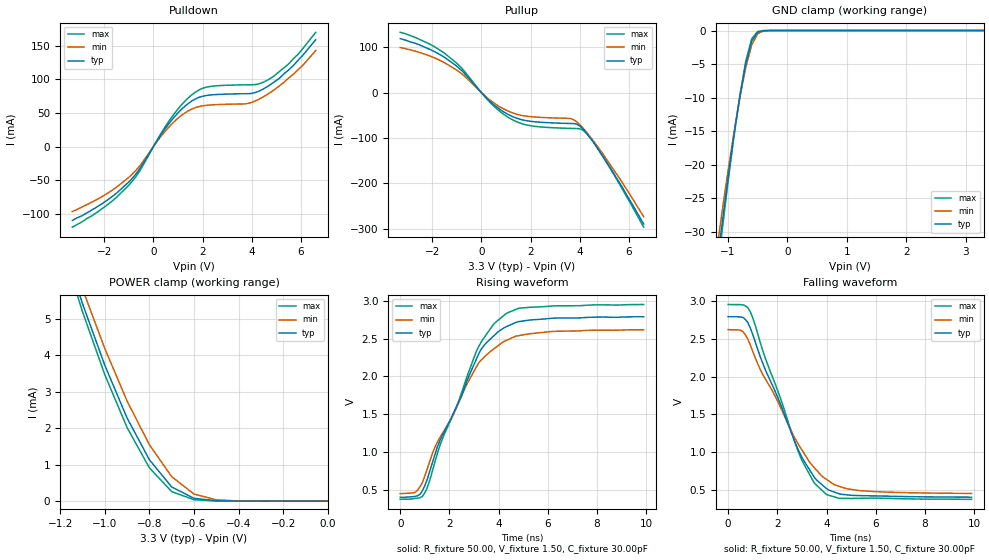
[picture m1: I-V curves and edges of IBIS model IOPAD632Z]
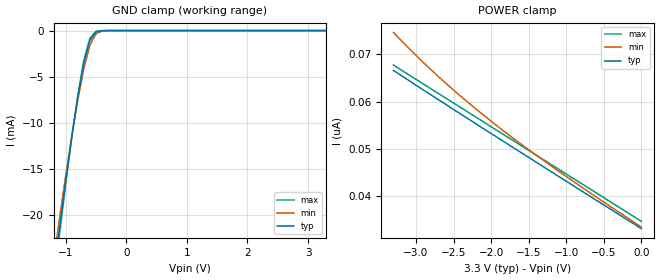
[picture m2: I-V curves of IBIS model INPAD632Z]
| IBIS file idt71v632z.ibs created by s2ibis2 version 1.1
| North Carolina State University Electronics Research Laboratory  1995
[IBIS ver]   2.1
[File name]   71v632z_pf.ibs
[File Rev]   1.1
[Date]   08/15/00
[Source]   Integrated Device Technology, Inc.
[Notes]   1. Temperatures: typ=25C, min=70C, max=0C 2. Cemos9_3v
   process. 3. Ramp rates based on 50 ohm load.
[Copyright]   Copyright 1998, Integrated Device Technology, Inc. Integrated
   Device Technology, Inc. ("IDT") hereby grants the user of this
   IBIS model a non-exclusive, nontransferable license to use
   this IBIS model under the following terms. The user is granted
   this license only to use the IBIS model and is not granted
   rights to sell, copy (except as needed to run the IBIS model),
   rent, lease or sub-license the IBIS model in whole or in part,
   or in modified form to anyone. The User may modify the IBIS
   model to suit its specific applications, but rights to
   derivative works and such modifications shall belong to IDT.
   This IBIS model is provided on an AS IS" basis and IDT makes
   absolutely no warranty with respect to the information
   contained herein. IDT DISCLAIMS AND CUSTOMER WAIVES ALL
   WARRANTIES, EXPRESS AND IMPLIED, INCLUDING WARRANTIES OF
   MERCHANTABILITY AND FITNESS FOR A PARTICULAR PURPOSE. THE
   ENTIRE RISK AS TO QUALITY AND PERFORMANCE IS WITH THE USER
   ACCORDINGLY, IN NO EVENT SHALL IDT BE LIABLE FOR ANY DIRECT OR
   INDIRECT DAMAGES, WHETHER IN CONTRACT OR TORT, INCLUDING ANY
   LOST PROFITS OR OTHER INCIDENTAL, CONSEQUENTIAL, EXEMPLARY, OR
   PUNITIVE DAMAGES ARISING OUT OF THE USE OR APPLICATION OF THE
   IBIS model. Further, IDT reserves the right to make changes
   without notice to any product herein to improve reliability,
   function, or design. IDT does not convey any license under
   patent rights or any other intellectual property rights,
   including those of third parties. IDT is not obligated to
   provide maintenance or support for the licensed IBIS model.
|   Component idt71V632Z
[Component]   idt71V632Z
[Manufacturer]   Integrated Device Technology
|   This component uses the 100 pin TQFP package (PF)
[Package]
| variable   typ   min   max
R_pkg   0.75   0.60   0.90
L_pkg   5.00nH   4.50nH   5.50nH
C_pkg   10.00fF   10.00fF   10.00fF
[Pin]  signal_name   model_name   R_pin   L_pin   C_pin
1   NC   NC
2   IO16   IOPAD632Z
3   IO17   IOPAD632Z
4   VDDQ   POWER
5   VSSQ   GND
6   IO18   IOPAD632Z
7   IO19   IOPAD632Z
8   IO20   IOPAD632Z
9   IO21   IOPAD632Z
10   VSSQ   GND
11   VDDQ   POWER
12   IO22   IOPAD632Z
13   IO23   IOPAD632Z
14   VDD   INPAD632Z
15   VDD   POWER
16   NC   NC
17   VSS   GND
18   IO24   IOPAD632Z
19   IO25   IOPAD632Z
20   VDDQ   POWER
21   VSSQ   GND
22   IO26   IOPAD632Z
23   IO27   IOPAD632Z
24   IO28   IOPAD632Z
25   IO29   IOPAD632Z
26   VSSQ   GND
27   VDDQ   POWER
28   IO30   IOPAD632Z
29   IO31   IOPAD632Z
30   NC   NC
31   LBO#   INPAD632Z
32   A5   INPAD632Z
33   A4   INPAD632Z
34   A3   INPAD632Z
35   A2   INPAD632Z
36   A1   INPAD632Z
37   A0   INPAD632Z
38   NC   NC
39   NC   NC
40   VSS   GND
41   VDD   POWER
42   NC   NC
43   NC   NC
44   A10   INPAD632Z
45   A11   INPAD632Z
46   A12   INPAD632Z
47   A13   INPAD632Z
48   A14   INPAD632Z
49   A15   INPAD632Z
50   NC   NC
51   NC   NC
52   IO0   IOPAD632Z
53   IO1   IOPAD632Z
54   VDDQ   POWER
55   VSSQ   GND
56   IO2   IOPAD632Z
57   IO3   IOPAD632Z
58   IO4   IOPAD632Z
59   IO5   IOPAD632Z
60   VSSQ   GND
61   VDDQ   POWER
62   IO6   IOPAD632Z
63   IO7   IOPAD632Z
64   ZZ   INPAD632Z
65   VDD   POWER
66   NC   NC
67   VSS   GND
68   IO8   IOPAD632Z
69   IO9   IOPAD632Z
70   VDDQ   POWER
71   VSSQ   GND
72   IO10   IOPAD632Z
73   IO11   IOPAD632Z
74   IO12   IOPAD632Z
75   IO13   IOPAD632Z
76   VSSQ   GND
77   VDDQ   POWER
78   IO14   IOPAD632Z
79   IO15   IOPAD632Z
80   NC   NC
81   A9   INPAD632Z
82   A8   INPAD632Z
83   ADV#   INPAD632Z
84   ADSP#   INPAD632Z
85   ADSC#   INPAD632Z
86   OE#   INPAD632Z
87   BWE#   INPAD632Z
88   GW#   INPAD632Z
89   CLK   INCLK632Z
90   VSS   GND
91   VDD   POWER
92   CS1#   INPAD632Z
93   BW1#   INPAD632Z
94   BW2#   INPAD632Z
95   BW3#   INPAD632Z
96   BW4#   INPAD632Z
97   CS0   INPAD632Z
98   CE#   INPAD632Z
99   A7   INPAD632Z
100   A6   INPAD632Z
| Models and submodels in the file (3): IOPAD632Z (I/O), INPAD632Z (Input), INCLK632Z (Input)
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| IOIN IOIN   dummy_model
| OE   OE   dummy_model
| POUT POUT   dummy_model
| COUT COUT   dummy_model
|   Model IOPAD632Z
[Model]   IOPAD632Z
Model_type   I/O
Polarity   Non-Inverting
Enable   Active-High
Vinl =  0.800V
Vinh =  2.000V
Vmeas =  1.500V
C_comp   3.00pF   NA   NA
[Temperature Range]   25.00   70.00   0.000
[Voltage Range]   3.30V   3.13V   3.46V
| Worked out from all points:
|   slope of the pulldown table from 0 to 0.495 V, typ, clamps not added: 18 ohm
|   slope of the pullup table from 0 to 0.495 V, typ, clamps not added: 19 ohm
|   GND clamp passes 1 mA (typ) near -0.56 V on its own axis
|   POWER clamp passes 1 mA (typ) near -0.78 V on its own axis
|   rising waveform, R_fixture 50.00, V_fixture 1.50, C_fixture 30.00pF: 20-80 % time 1.88ns typ, 1.99ns min, 1.83ns max; typ from 0.402 V to 2.79 V
|   falling waveform, R_fixture 50.00, V_fixture 1.50, C_fixture 30.00pF: 20-80 % time 1.84ns typ, 2.09ns min, 1.68ns max; typ from 2.79 V to 0.405 V
[Pulldown]
| voltage   I(typ)   I(min)   I(max)
-3.3V     -110mA     -96.8mA    -120mA
-1.9V     -80.34mA   -70.29mA   -87.42mA
-1V       -52.66mA   -45.75mA   -57.44mA
-600mV    -35.41mA   -30.69mA   -38.63mA
700mV     37.46mA    31.83mA    41.5mA
1.2V      57.39mA    47.94mA    64.43mA
1.6V      68.62mA    56.39mA    78.1mA
2.3V      76.66mA    61.8mA     89.38mA
3.8V      78.66mA    63.9mA     91.88mA
4.5V      86.32mA    74.69mA    96.28mA
5.5V      114mA      102mA      123mA
6.6V      159mA      143mA      170mA
[Pullup]
| voltage   I(typ)   I(min)   I(max)
-3.3V     119mA      99.42mA    133mA
-2.1V     95.52mA    80.86mA    107mA
-1.5V     77.88mA    66.15mA    86.84mA
-800mV    48.45mA    41.43mA    53.79mA
400mV     -21.63mA   -18.48mA   -24.22mA
1.2V      -51.24mA   -43.4mA    -58.1mA
2V        -63.41mA   -53.08mA   -73.13mA
3.6V      -68.15mA   -57.15mA   -78.99mA
4V        -73.61mA   -70.75mA   -79.92mA
4.3V      -91.05mA   -88.93mA   -91.73mA
4.7V      -121mA     -117mA     -121mA
6.6V      -290mA     -274mA     -297mA
[GND_clamp]
| voltage   I(typ)   I(min)   I(max)
-3.3V     -218mA     -200mA     -230mA
-1.2V     -36.17mA   -33.59mA   -37.83mA
-1.1V     -28.94mA   -27.15mA   -30.08mA
-1V       -22.07mA   -21.03mA   -22.73mA
-900mV    -15.67mA   -15.31mA   -15.89mA
-800mV    -9.874mA   -10.07mA   -9.724mA
-700mV    -4.961mA   -5.537mA   -4.586mA
-600mV    -1.581mA   -2.168mA   -1.255mA
-500mV    -240uA     -482uA     -146uA
-400mV    -20.26uA   -61.48uA   -9.329uA
-300mV    -1.243uA   -5.894uA   -417nA
3.3V      33.12nA    55.61nA    33.01nA
[POWER_clamp]
| voltage   I(typ)   I(min)   I(max)
-3.3V     68.19mA    63.28mA    71.61mA
-1.2V     7.321mA    7.63mA     7.168mA
-1.1V     5.426mA    5.83mA     5.205mA
-1V       3.734mA    4.192mA    3.474mA
-900mV    2.282mA    2.748mA    2.019mA
-800mV    1.135mA    1.547mA    914uA
-700mV    390uA      672uA      261uA
-600mV    76.61uA    194uA      39.03uA
-500mV    9.431uA    35.28uA    3.792uA
-400mV    942nA      4.932uA    313nA
0V        33.12nA    33.67nA    34.67nA
[Ramp]
| variable   typ   min   max
dV/dt_r   1.37/1.48n   1.22/1.65n   1.50/1.35n
dV/dt_f   1.42/1.59n   1.27/1.89n   1.54/1.40n
R_load = 50.00
[Rising Waveform]
R_fixture = 50.00
V_fixture = 1.50
C_fixture = 30.00pF
R_dut = 0.75
L_dut = 0.10nH
C_dut = 0.53pF
| time   V(typ)   V(min)   V(max)
0s        402mV      451mV      375mV
600ps     414mV      466mV      386mV
1ns       556mV      684mV      460mV
1.6ns     1.142V     1.184V     1.075V
2.3ns     1.61V      1.597V     1.607V
3.1ns     2.231V     2.128V     2.333V
3.4ns     2.407V     2.252V     2.508V
4.2ns     2.638V     2.459V     2.803V
5.3ns     2.747V     2.565V     2.915V
9.9ns     2.788V     2.616V     2.95V
[Falling Waveform]
R_fixture = 50.00
V_fixture = 1.50
C_fixture = 30.00pF
R_dut = 0.75
L_dut = 0.10nH
C_dut = 0.53pF
| time   V(typ)   V(min)   V(max)
0s        2.791V     2.62V      2.952V
600ps     2.782V     2.593V     2.947V
900ps     2.642V     2.417V     2.855V
1.3ns     2.267V     2.098V     2.456V
2.9ns     999mV      1.081V     968mV
3.5ns     671mV      797mV      593mV
4ns       519mV      640mV      440mV
4.4ns     463mV      561mV      401mV
5.3ns     427mV      494mV      391mV
9.9ns     405mV      455mV      377mV
|   Model INPAD632Z
[Model]   INPAD632Z
Model_type   Input
Vinl =  0.800V
Vinh =  2.000V
Vmeas =  1.500V
C_comp   3.00pF   NA   NA
[Temperature Range]   25.00   70.00   0.000
[Voltage Range]   3.30V   3.13V   3.46V
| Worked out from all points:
|   GND clamp passes 1 mA (typ) near -0.59 V on its own axis
[GND_clamp]
| voltage   I(typ)   I(min)   I(max)
-3.3V     -154mA     -142mA     -161mA
-1.2V     -26.63mA   -25.02mA   -27.64mA
-1.1V     -21.34mA   -20.27mA   -22.01mA
-1V       -16.3mA    -15.73mA   -16.64mA
-900mV    -11.56mA   -11.46mA   -11.6mA
-800mV    -7.239mA   -7.529mA   -7.033mA
-700mV    -3.571mA   -4.11mA    -3.224mA
-600mV    -1.088mA   -1.583mA   -820uA
-500mV    -157uA     -346uA     -87.87uA
-400mV    -13.22uA   -44.52uA   -5.567uA
-300mV    -814nA     -4.323uA   -249nA
3.3V      33.1nA     35.18nA    33.01nA
[POWER_clamp]
| voltage   I(typ)   I(min)   I(max)
-3.3V     66.6nA     74.65nA    67.74nA
-3V       63.48nA    69.79nA    64.72nA
-2.7V     60.39nA    65.28nA    61.71nA
-2.3V     56.3nA     59.73nA    57.69nA
-1.9V     52.23nA    54.61nA    53.68nA
-1.1V     44.15nA    45.26nA    45.67nA
0V        33.1nA     33.44nA    34.66nA
